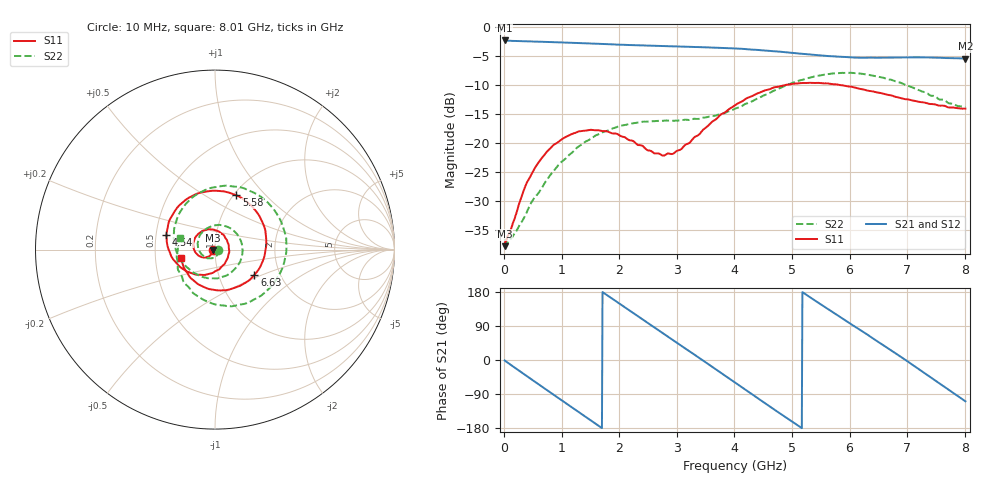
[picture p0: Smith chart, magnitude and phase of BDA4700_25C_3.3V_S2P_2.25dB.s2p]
!Agilent Technologies,E5071B,MY42404982,A.09.10
!Date: Mon Oct 20 18:03:55 2025
!Data & Calibration Information:
!Freq	S11:SOLT2(ON)	S21:SOLT2(ON)	S12:SOLT2(ON)	S22:SOLT2(ON)
# Hz S RI R 50
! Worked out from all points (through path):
!   801 points, 10 MHz to 8.01 GHz, reference 50 ohm
!   highest |S21| = -2.37 dB at 10 MHz (marker M1); lowest = -5.5 dB at 8.01 GHz (marker M2)
!   group delay of S21, straight-line fit = 286 ps
!   lowest |S11| = -37.8 dB at 10 MHz (marker M3), VSWR 1.03, Z = 48.7 - j0.171 ohm
!   |S11| at or under -10 dB: start of sweep to 4.907 GHz; 5.8 GHz to end of sweep
!   |S22| runs from -37.4 to -7.9 dB; largest |S21 - S12| = 0.0086
!   S11 on the Smith chart (normalised r, x): 10 MHz: 0.97, -0.00; 4.54 GHz: 0.57, +0.10; 5.58 GHz: 1.03, +0.70; 6.63 GHz: 1.48, -0.44; 8.01 GHz: 0.68, -0.07
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1e7  -0.0127 -0.00176  0.7615 -0.0163  0.7614 -0.0169  0.0147 -0.0015
3.3e8  -0.0234 -0.0293  0.6107 -0.4355  0.6105 -0.4358  0.0167 -0.014
7.2e8  -0.068 -0.0436  0.1686 -0.7203  0.169 -0.7205  -0.00734 -0.0454
1.02e9  -0.1066 -0.0185  -0.2305 -0.6943  -0.2306 -0.6944  -0.0553 -0.0423
1.35e9  -0.1203 0.0373  -0.5771 -0.4336  -0.5773 -0.434  -0.0951 0.0167
1.64e9  -0.0938 0.0873  -0.708 -0.0817  -0.708 -0.0816  -0.077 0.0897
1.92e9  -0.0431 0.1121  -0.6495 0.2709  -0.6498 0.271  -0.00513 0.1343
2.32e9  0.0353 0.089  -0.3035 0.6217  -0.3028 0.6219  0.115 0.0951
2.68e9  0.0763 0.0265  0.1332 0.6707  0.1321 0.6703  0.1527 -0.0224
3.36e9  0.0138 -0.1144  0.6606 0.0975  0.6618 0.0974  -0.00716 -0.1599
3.67e9  -0.0724 -0.1404  0.6036 -0.2668  0.603 -0.2686  -0.1028 -0.1367
4.01e9  -0.1817 -0.1063  0.3301 -0.5596  0.331 -0.5587  -0.1843 -0.0667
4.54e9  -0.2709 0.0833  -0.2631 -0.5651  -0.262 -0.5661  -0.224 0.1302
4.94e9  -0.1921 0.253  -0.5489 -0.2398  -0.5485 -0.2429  -0.1206 0.2951
5.35e9  -0.000116 0.3277  -0.5455 0.1792  -0.5467 0.1762  0.1081 0.351
5.58e9  0.1188 0.3023  -0.4228 0.3693  -0.4233 0.369  0.245 0.3017
6.09e9  0.2806 0.1056  0.0165 0.5418  0.0181 0.5442  0.3981 0.0157
6.63e9  0.2198 -0.1397  0.4465 0.3064  0.4472 0.3053  0.2354 -0.2684
6.68e9  0.2038 -0.1577  0.4708 0.2661  0.4727 0.2652  0.2074 -0.284
7.25e9  -0.0193 -0.2228  0.4753 -0.2649  0.4752 -0.2654  -0.0935 -0.2608
7.63e9  -0.1386 -0.156  0.1936 -0.5022  0.1932 -0.5028  -0.2063 -0.1121
8.01e9  -0.1911 -0.0474  -0.1731 -0.5021  -0.1713 -0.503  -0.1942 0.0619
